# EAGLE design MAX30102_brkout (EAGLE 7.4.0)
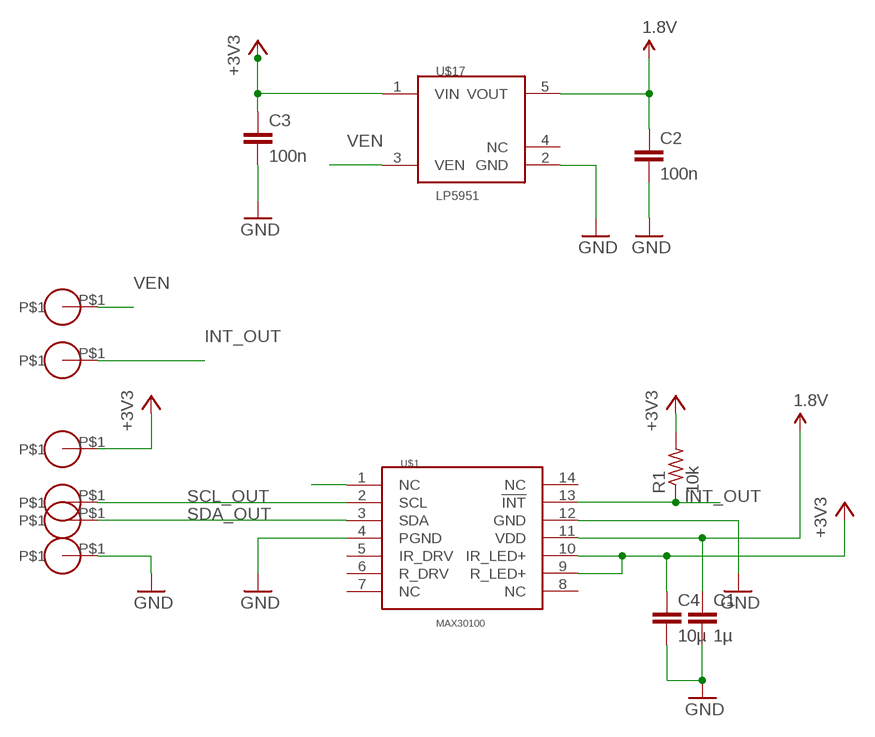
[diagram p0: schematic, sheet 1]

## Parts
C1  1µ  C-EUC0402  [C0402]
C2  100n  C-EUC0402  [C0402]
C3  100n  C-EUC0402  [C0402]
C4  10µ  C-EUC0603  [C0603]
R1  10k  R-US_R0402  [R0402]
U$1  MAX30100  [OESIP-14]
U$3  MINIPAD  [MINIPAD]
U$4  MINIPAD  [MINIPAD]
U$5  MINIPAD  [MINIPAD]
U$6  MINIPAD  [MINIPAD]
U$8  MINIPAD  [MINIPAD]
U$9  MINIPAD  [MINIPAD]
U$17  LP5951  [SC70-5]

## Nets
1.8V: C1.1 C2.1 U$1.11(VDD) U$17.5(VOUT)
+3V3: C3.1 C4.1 R1.2 U$1.9(R_LED+) U$1.10(IR_LED+) U$4.P$1 U$17.1(VIN)
GND: C1.2 C2.2 C3.2 C4.2 U$1.4(PGND) U$1.12(GND) U$8.P$1 U$17.2(GND)
INT_OUT: R1.1 U$1.13(!INT) U$3.P$1
N$2: U$1.1(NC)
SCL_OUT: U$1.2(SCL) U$5.P$1
SDA_OUT: U$1.3(SDA) U$6.P$1
VEN: U$9.P$1 U$17.3(VEN)
Unconnected: U$1.5(IR_DRV) U$1.6(R_DRV) U$1.7(NC) U$1.8(NC) U$1.14(NC) U$17.4(NC)

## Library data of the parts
C1-C4 = rcl:C-EU: CAPACITOR, European symbol
R1 = rcl:R-US_: RESISTOR, American symbol
U$1 = circuitects:MAX30100
U$3-U$6 U$8 U$9 = minipad:MINIPAD
U$17 = circuitects:LP5951

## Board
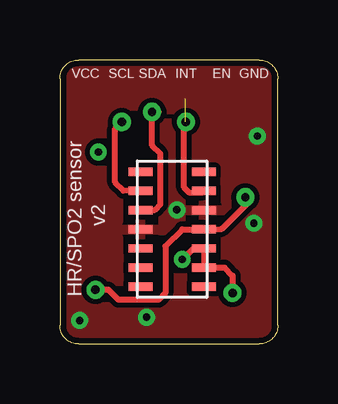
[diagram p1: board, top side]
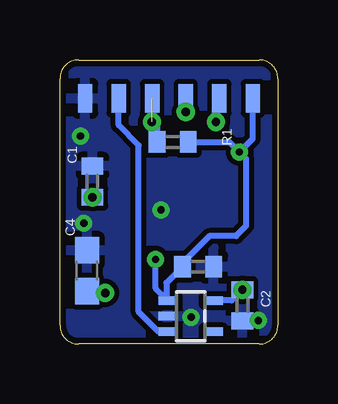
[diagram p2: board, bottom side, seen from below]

Size 9.1 x 11.85 mm. Coordinates in mm from the lower left corner, seen from the top.
Outline: 0.78,0 8.32,0 arc90 9.1,0.77 9.1,11.07 arc90 8.32,11.85 0.78,11.85 arc90 0,11.07 0,0.77 arc90 0.78,0
Copper layers (1*16): Top 0.035mm / dielectric 1.5mm / Bottom 0.035mm
Design rules "default *": minimum track width 10mil, minimum drill 24mil, track to track 8mil, track to pad 8mil, pad to pad 8mil, via to via 8mil, smd to smd 8mil, copper to edge 10mil, drill to drill 8mil, minimum pad ring 10mil, minimum via ring 8mil, stop-mask expansion 4mil, vias tented up to drill 20mil, thermal gap 10mil

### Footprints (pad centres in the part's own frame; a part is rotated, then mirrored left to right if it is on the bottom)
C0402 = smd 0.7 x 0.9: 1 -0.65,0; 2 0.65,0
C0603 = smd 1.1 x 1: 1 -0.85,0; 2 0.85,0
R0402 = smd 0.7 x 0.9: 1 -0.65,0; 2 0.65,0
OESIP-14 = smd 1 x 0.35: 1 -1.325,2.4; 2 -1.325,1.6; 3 -1.325,0.8; 4 -1.325,0; 5 -1.325,-0.8; 6 -1.325,-1.6; 7 -1.325,-2.4; 8 1.325,-2.4; 9 1.325,-1.6; 10 1.325,-0.8; 11 1.325,0; 12 1.325,0.8; 13 1.325,1.6; 14 1.325,2.4
MINIPAD = smd 1.2 x 0.6: P$1 0,0
SC70-5 = smd 0.35 x 0.8: 1 -0.65,-0.95; 2 0,-0.95; 3 0.65,-0.95; 4 0.65,0.95; 5 -0.65,0.95

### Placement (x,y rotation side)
C1  7.74,6.77 90 bottom
C2  1.48,1.61 270 bottom
C3  3.33,3.22 0 bottom
C4  7.96,3.06 90 bottom
R1  4.39,8.43 0 bottom
U$1  4.68,4.79 0 top
U$3  5.25,10.24 90 bottom
U$4  1.05,10.24 90 bottom
U$5  2.44,10.24 90 bottom
U$6  3.84,10.24 90 bottom
U$8  8.04,10.24 90 bottom
U$9  6.64,10.24 90 bottom
U$17  3.64,1.16 270 bottom

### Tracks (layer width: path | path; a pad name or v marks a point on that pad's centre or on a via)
1.8V  (via drill 0.35)
  Top 0.254: C1.1 7.88,5.93 6.75,4.8 U$1.11 5.1,4.79 4.41,4.08 4.41,2.12 4.12,1.85 2.44,1.85 2.03,2.26 C2.1
  Bottom 0.254: C2.1 1.93,1.81 U$17.5
  other vias: 7.74,6.12 1.48,2.26
+3V3  (via drill 0.3, 0.35)
  Top 0.254: v5.1,3.53 5.56,3.99 U$1.10 U$1.9 6.87,3.18 7.21,2.85 v7.21,2.12 | v1.6,8.01 1.6,8.14
  Bottom 0.254: v1.6,8.01 1.32,7.72 1.32,4.92 1.75,4.5 2.86,4.5 3.98,3.39 C3.1 4.65,2.55 4.65,1.88 | R1.2 2.03,8.43 v1.6,8.01 | U$17.1 4.65,1.88 | 4.65,1.88 5.1,2.33 v5.1,3.53 | v7.21,2.12 7.88,2.12 C4.1 | v1.6,8.01 1.05,8.56 U$4.P$1
GND  (via drill 0.3)
  other vias: 0.82,0.98 8.24,8.68 8.1,5.04 4.88,5.6 3.62,1.12
  pour Bottom: -2.92,13.32 -2.92,-3.73 10.65,-3.73 10.65,13.32
  pour Top: -2.14,12.94 -2.14,-2.95 9.87,-2.95 9.87,12.94
INT_OUT  (via drill 0.35)  (1 unrouted)
  Top 0.254: U$1.13 5.95,6.33 5.38,6.33 5.18,6.53 5.18,9.19 v5.25,9.27
  Bottom 0.254: v5.25,9.27 5.04,9.05 R1.1
SCL_OUT  (via drill 0.35)
  Top 0.254: U$1.2 2.65,6.4 2.3,6.74 2.3,8.98 v2.58,9.27
  Bottom 0.254: v2.58,9.27 2.58,10.11 U$5.P$1
SDA_OUT  (via drill 0.35)
  Top 0.254: U$1.3 3.96,5.6 4.19,5.83 4.19,7.94 3.84,8.29 v3.84,9.69 4.12,9.69
  Bottom 0.254: v3.84,9.69 U$6.P$1
VEN
  Bottom 0.254: U$17.3 4.98,0.51 5.8,1.34 5.8,8.29 6.64,9.12 U$9.P$1

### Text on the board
tPlace: VCC | SCL | SDA | INT | EN | GND | v2 | HR/SPO2 sensor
